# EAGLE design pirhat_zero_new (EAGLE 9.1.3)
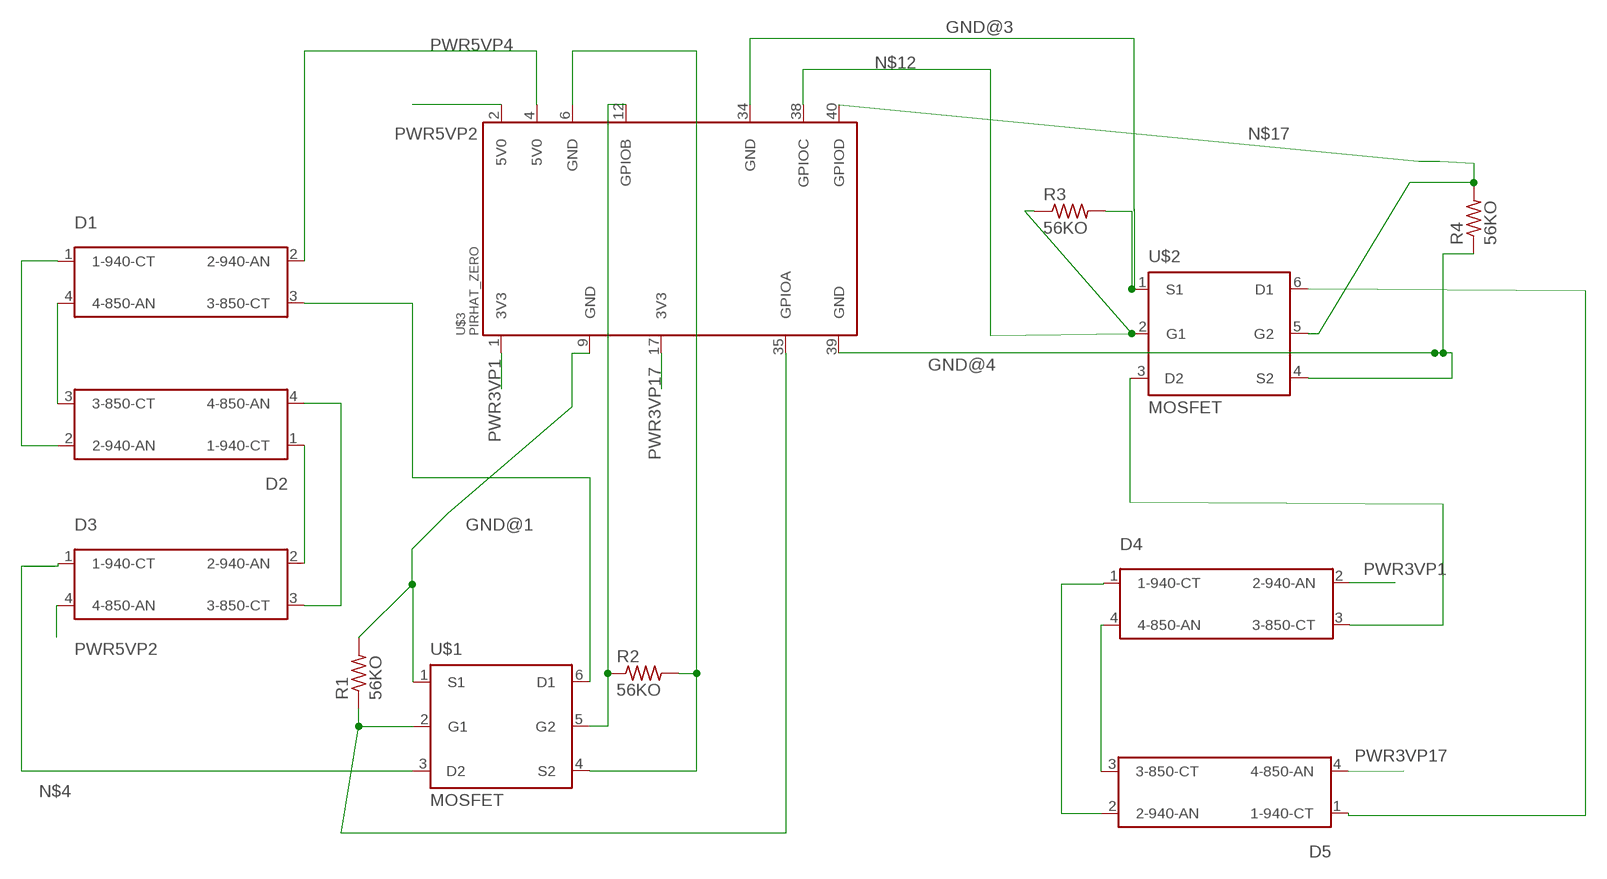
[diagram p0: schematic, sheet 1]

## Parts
D1  LED_SFH7252  [LED_SFH7252]
D2  LED_SFH7252  [LED_SFH7252]
D3  LED_SFH7252  [LED_SFH7252]
D4  LED_SFH7252  [LED_SFH7252]
D5  LED_SFH7252  [LED_SFH7252]
R1  56KO  TE_56KO_RESIST_CRG1206F56K  [TE_56KO_RESIST_CRG1206F56K]
R2  56KO  TE_56KO_RESIST_CRG1206F56K  [TE_56KO_RESIST_CRG1206F56K]
R3  56KO  TE_56KO_RESIST_CRG1206F56K  [TE_56KO_RESIST_CRG1206F56K]
R4  56KO  TE_56KO_RESIST_CRG1206F56K  [TE_56KO_RESIST_CRG1206F56K]
U$1  MOSFET  ON_MOSFET_NTJD4001NT1GRPI  [ON_MOSFET_NTJD4001NT1G]
U$2  MOSFET  ON_MOSFET_NTJD4001NT1GRPI  [ON_MOSFET_NTJD4001NT1G]
U$3  PIRHAT_ZERO  [PIRHAT_ZERO]

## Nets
GND@1: R1.2 U$1.1(S1) U$3.9(GND)
GND@2: R2.2 U$1.4(S2) U$3.6(GND)
GND@3: R3.2 U$2.1(S1) U$3.34(GND)
GND@4: R4.1 U$2.4(S2) U$3.39(GND)
N$1: D1.3(3-850-CT) U$1.6(D1)
N$2: D1.1(1-940-CT) D2.2(2-940-AN)
N$3: D2.1(1-940-CT) D3.2(2-940-AN)
N$4: D3.1(1-940-CT) U$1.3(D2)
N$5: R2.1 U$1.5(G2) U$3.12(GPIOB)
N$6: R1.1 U$1.2(G1) U$3.35(GPIOA)
N$7: D4.1(1-940-CT) D5.2(2-940-AN)
N$8: D2.4(4-850-AN) D3.3(3-850-CT)
N$9: D1.4(4-850-AN) D2.3(3-850-CT)
N$10: D4.4(4-850-AN) D5.3(3-850-CT)
N$11: D5.1(1-940-CT) U$2.6(D1)
N$12: R3.1 U$2.2(G1) U$3.38(GPIOC)
N$13: D4.3(3-850-CT) U$2.3(D2)
N$17: R4.2 U$2.5(G2) U$3.40(GPIOD)
PWR3VP1: D4.2(2-940-AN) U$3.1(3V3)
PWR3VP17: D5.4(4-850-AN) U$3.17(3V3)
PWR5VP2: D3.4(4-850-AN) U$3.2(5V0)
PWR5VP4: D1.2(2-940-AN) U$3.4(5V0)

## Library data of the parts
D1-D5 = pirhat_zero:LED_SFH7252: Osram SFH 7252 Infrared Emitter (850 nm) and Infrared Emitter (940 nm)
R1-R4 = pirhat_zero:TE_56KO_RESIST_CRG1206F56K: Res Thick Film 1206 56K Ohm 1% 0.25W(1/4W) ¯100ppm/®C Molded SMD T/R; AVAILABILITY: Unavailable; COMMENT: 1623536-1; DESCRIPTION: CRG1206 1% 56K; EU_ROHS_COMPLIANCE: Compliant with Exemptions; MF: TE Connectivity; MP: CRG1206F56K; PACKAGE: 1206; POWER_RATING: .25 W; PRICE: None; RESISTANCE: 56K; TE_PURCHASE_URL: https://www.te.com/usa-en/product-1623536-1.html?te_bu=Cor&te_type=disp&te_campaign=seda_glo_cor-seda-global-disp-prtnr-fy19-seda-model-bom-cta_sma-317_1&elqCampaignId=32493; TOLERANCE: 1%; VOLTAGE_RATING: 200 V
U$1 U$2 = pirhat_zero:ON_MOSFET_NTJD4001NT1G
U$3 = pirhat_zero:PIRHAT_ZERO

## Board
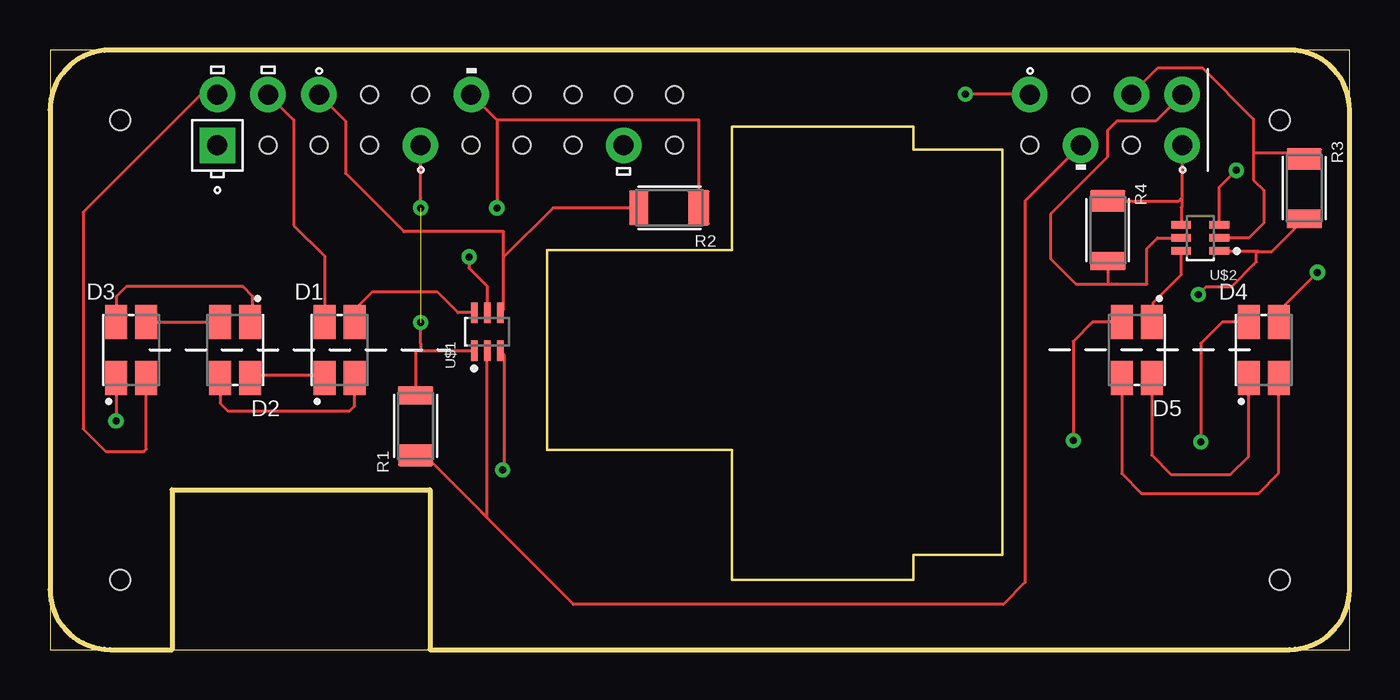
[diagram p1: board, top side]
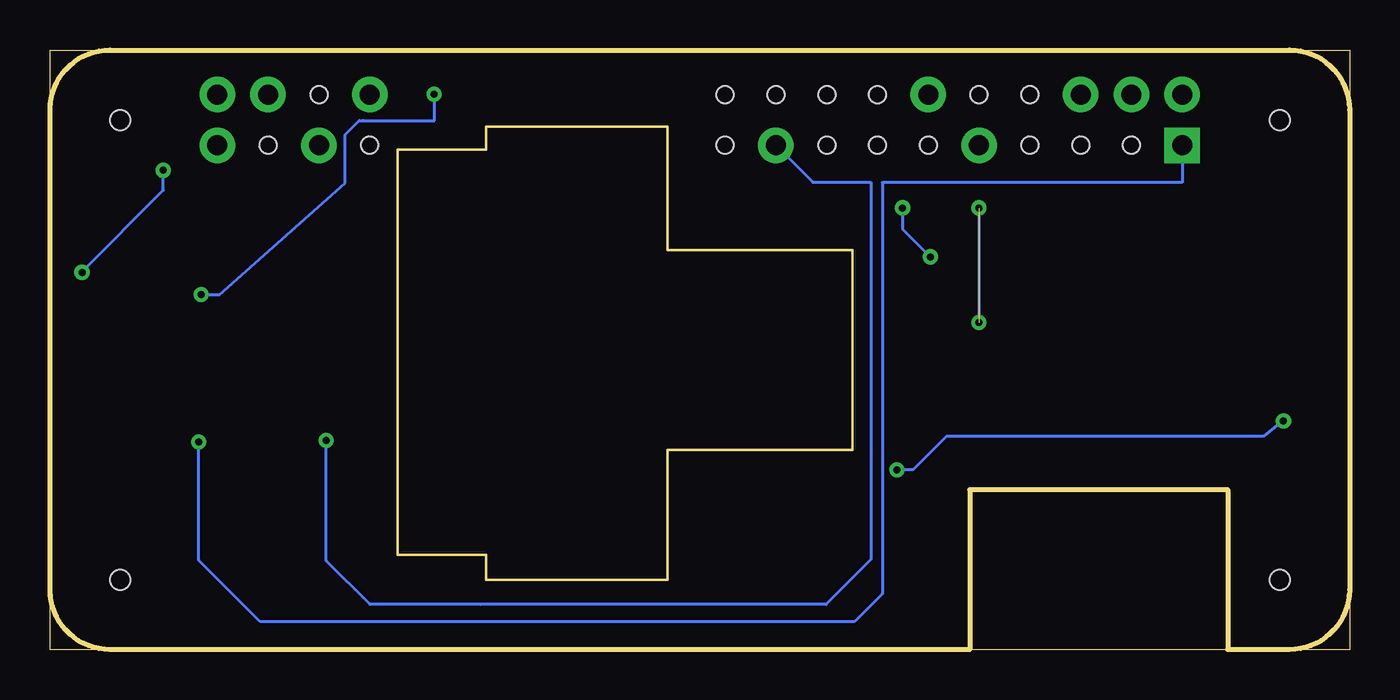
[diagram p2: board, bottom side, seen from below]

Size 65 x 30 mm. Coordinates in mm from the lower left corner, seen from the top.
Outline: 0,0 65,0 65,30 0,30 0,0
Copper layers (1*16): Top 0.035mm / dielectric 1.5mm / Bottom 0.035mm
Design rules "pirhat *": minimum track width 6mil, minimum drill 0.35mm, track to track 6mil, track to pad 6mil, pad to pad 6mil, via to via 6mil, smd to smd 6mil, copper to edge 0.7mm, drill to drill 0.01mm, minimum pad ring 10mil, minimum via ring 8mil, stop-mask expansion 4mil, vias tented up to drill 0mil, thermal gap 10mil

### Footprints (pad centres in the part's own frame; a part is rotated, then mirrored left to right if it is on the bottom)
LED_SFH7252 = smd 1.1 x 1.7: 1 -0.75,-1.4; 2 -0.75,1.4; 3 0.75,1.4; 4 0.75,-1.4
TE_56KO_RESIST_CRG1206F56K = smd 1.09 x 1.77: 1 -1.465,0 | smd 0.94 x 1.77: 2 1.54,0
ON_MOSFET_NTJD4001NT1G = smd 1.02 x 0.36: 1 -0.955,0.65; 2 -0.955,0; 3 -0.955,-0.65; 4 0.955,-0.65; 5 0.955,0; 6 0.955,0.65
PIRHAT_ZERO = drill 1 pad 1.778 square: 1 8.37,25.23 | drill 1 pad 1.778: 2 8.37,27.77; 4 10.91,27.77; 6 13.45,27.77; 9 18.53,25.23; 12 21.07,27.77; 17 28.69,25.23; 34 49.01,27.77; 35 51.55,25.23; 38 54.09,27.77; 39 56.63,25.23; 40 56.63,27.77 | hole 1: 3.5,3.5; 3.5,26.5; 61.5,3.5; 61.5,26.5 | hole 0.85: 54.09,25.23; 51.55,27.77; 31.23,25.23; 26.15,25.23; 15.99,27.77; 49.01,25.23; 23.61,25.23; 15.99,25.23; 13.45,25.23; 10.91,25.23; 21.07,25.23; 23.61,27.77; 28.69,27.77; 31.23,27.77; 26.15,27.77; 18.53,27.77

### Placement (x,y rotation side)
D1  14.48,14.99 0 top
D2  9.27,14.99 180 top
D3  4.06,14.99 0 top
D4  60.71,14.99 0 top
D5  54.36,14.99 180 top
R1  18.29,11.18 90 top
R2  30.99,22.1 180 top
R3  62.74,23.09 270 top
R4  52.91,20.98 270 top
U$1  21.87,15.9 90 top
U$2  57.53,20.6 180 top
U$3  0,0 0 top

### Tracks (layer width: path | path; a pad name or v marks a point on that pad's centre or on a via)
GND@1  (via drill 0.35)  (1 unrouted)
  Top 0.152: 18.54,14.95 18.54,15.3 v18.54,16.36 | 18.54,22.61 v18.54,22.1 18.54,25.23 U$3.9 | U$1.1 18.54,14.95 | 18.54,14.95 18.29,14.95 R1.2
  Bottom 0.152: v18.54,22.1 v18.54,16.36
GND@2
  Top 0.152: U$3.6 14.78,26.44 14.78,23.83 17.7,20.9 22.7,20.9 22.7,19.63 | 22.58,16.91 U$1.4 22.7,17.03 22.7,19.63 | R2.2 25.16,22.1 22.7,19.63
GND@3  (via drill 0.35)
  Top 0.152: v45.8,27.79 48.99,27.79 U$3.34 | R3.2 61.11,19.92 60.45,19.92 | U$2.1 60.43,19.95 60.45,19.92 | 60.45,19.92 60.35,19.92 60.35,19.41 60.22,19.28 59.08,18.14 57.81,18.14 v57.43,17.75
  Bottom 0.152: v57.43,17.75 56.52,17.75 50.24,23.34 50.24,25.76 49.53,26.47 49.34,26.47 45.77,26.47 45.77,27.76 v45.8,27.79
GND@4
  Top 0.152: 56.61,22.61 56.61,25.21 U$3.39 | 56.61,22.61 56.61,22.15 56.58,22.11 U$2.4 | R4.1 56.45,22.45 56.61,22.61
N$1
  Top 0.152: D1.3 15.23,17.01 16.13,17.91 19.36,17.91 20.41,16.86 U$1.6
N$2
  Top 0.152: D1.1 13.86,13.72 10.02,13.72 D2.2
N$3
  Top 0.152: D3.2 3.31,17.66 3.81,18.16 9.65,18.16 10.15,17.66 10.15,16.51 D2.1
N$4  (via drill 0.35)
  Top 0.152: D3.1 3.31,11.44 v3.3,11.43 | U$1.3 22.73,14.73 22.73,9.09 v22.63,8.99
  Bottom 0.152: v3.3,11.43 3.35,11.44 4.32,10.67 20.16,10.67 21.83,8.99 v22.63,8.99
N$5  (via drill 0.35)
  Top 0.152: U$3.12 22.35,26.49 | 22.35,26.49 v22.35,22.1 | U$1.5 21.87,18.18 20.95,19.09 v20.95,19.65 | R2.1 32.45,26.49 22.35,26.49
  Bottom 0.152: v20.95,19.65 22.35,21.05 v22.35,22.1
N$6
  Top 0.152: U$3.35 48.77,22.45 48.77,3.35 47.68,2.26 26.19,2.26 21.59,6.86 21.59,6.88 | 21.59,6.88 21.87,6.6 U$1.2 | R1.1 18.15,9.58 18.9,9.58 21.59,6.88
N$7
  Top 0.152: D5.2 55.11,9.72 56.07,8.76 59.04,8.76 59.96,9.67 D4.1
N$8
  Top 0.152: D3.3 D2.4
N$9
  Top 0.152: D2.3 8.52,12.31 8.89,11.94 14.99,11.94 15.24,12.19 15.24,13.57 D1.4
N$10
  Top 0.152: D5.3 53.61,8.8 54.59,7.82 60.45,7.82 61.46,8.83 D4.4
N$11
  Top 0.152: D5.1 55.18,16.46 55.18,17.36 56.58,18.76 U$2.6
N$12
  Top 0.152: 60.2,24.87 60.2,26.54 57.66,29.08 55.4,29.08 U$3.38 | U$2.2 59.97,20.6 60.71,21.34 60.71,22.99 60.2,23.5 60.2,24.87 | 60.2,24.87 62.42,24.87 R3.1
N$13  (via drill 0.35)
  Top 0.152: D4.3 61.46,16.93 v63.4,18.87 | v59.33,23.98 58.49,23.13 U$2.3
  Bottom 0.152: v59.33,23.98 59.33,22.99 63.4,18.92 v63.4,18.87
N$17
  Top 0.152: 56.54,20.63 U$2.5 55.4,20.6 54.86,20.07 54.86,18.29 53.34,18.29 53.11,18.29 52.91,18.29 | U$3.40 55.31,26.45 53.37,26.45 52.89,25.96 52.89,24.64 50.04,21.79 50.04,19.56 51.31,18.29 52.91,18.29 | R4.2 52.91,18.29
PWR3VP1  (via drill 0.35)
  Top 0.152: D4.2 58.63,16.39 57.56,15.32 v57.56,10.39
  Bottom 0.152: U$3.1 8.37,23.37 23.37,23.37 23.37,2.79 24.77,1.4 54.48,1.4 57.56,4.47 v57.56,10.39
PWR3VP17  (via drill 0.35)
  Top 0.152: D5.4 52.15,16.39 51.18,15.42 v51.18,10.46
  Bottom 0.152: U$3.17 26.84,23.38 23.94,23.38 23.94,4.51 26.19,2.26 43.49,2.26 49,2.26 51.18,4.45 v51.18,10.46
PWR5VP2
  Top 0.152: U$3.2 7.54,27.77 1.65,21.89 1.65,11.05 2.79,9.91 4.69,9.91 4.81,10.03 D3.4
PWR5VP4
  Top 0.152: U$3.4 12.19,26.49 12.19,21.22 13.73,19.69 D1.2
